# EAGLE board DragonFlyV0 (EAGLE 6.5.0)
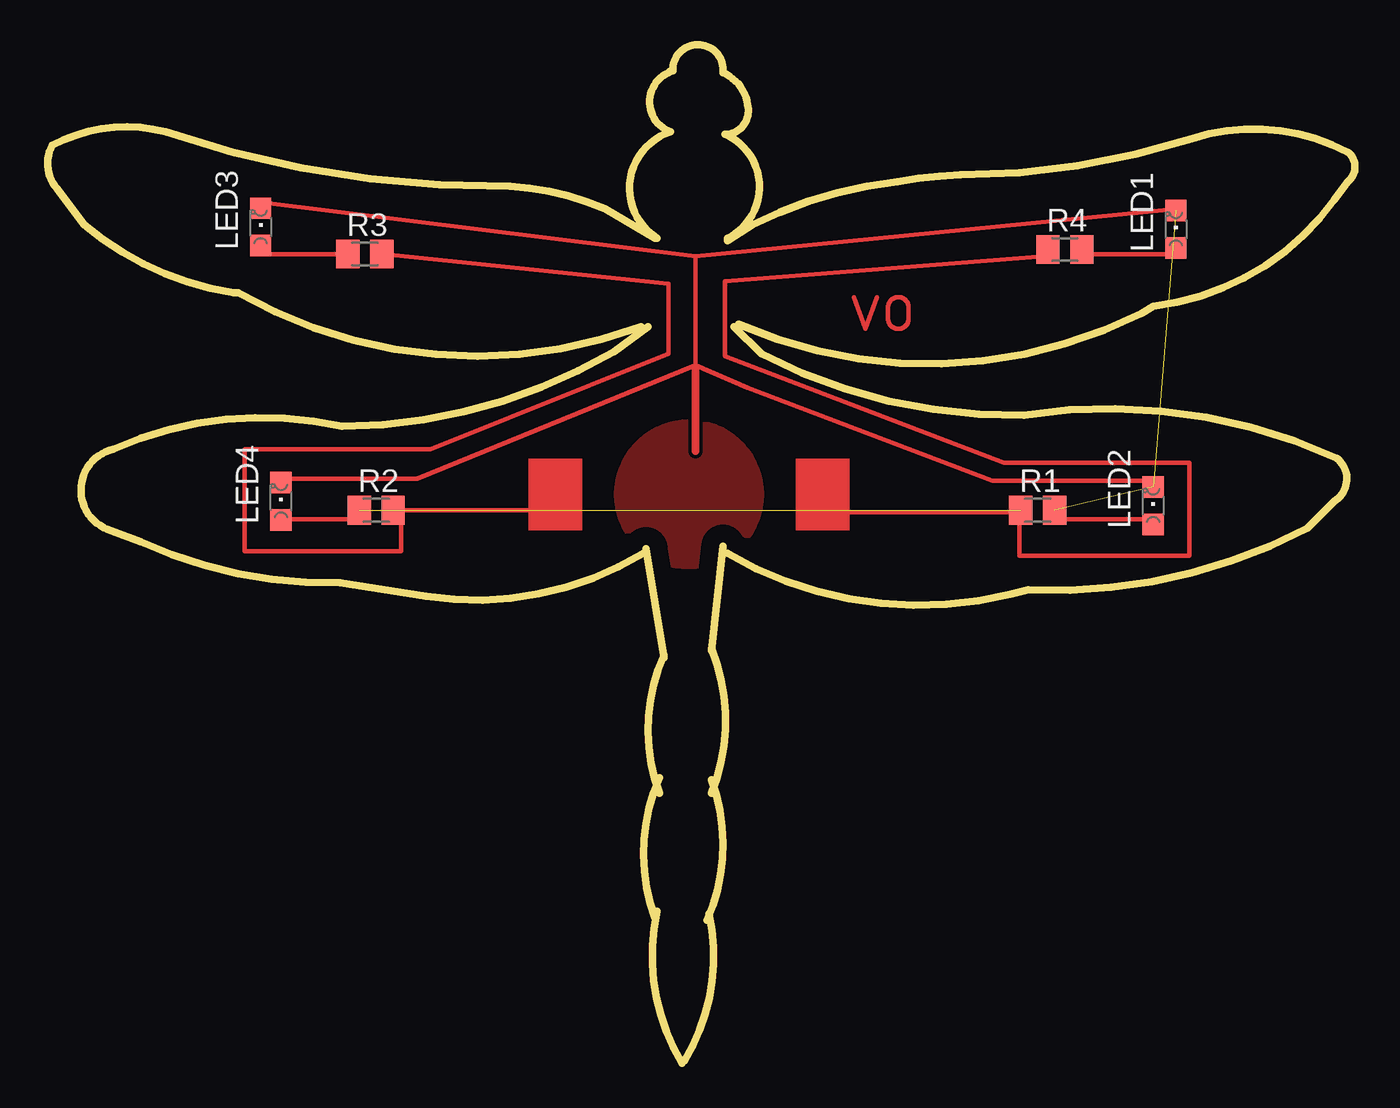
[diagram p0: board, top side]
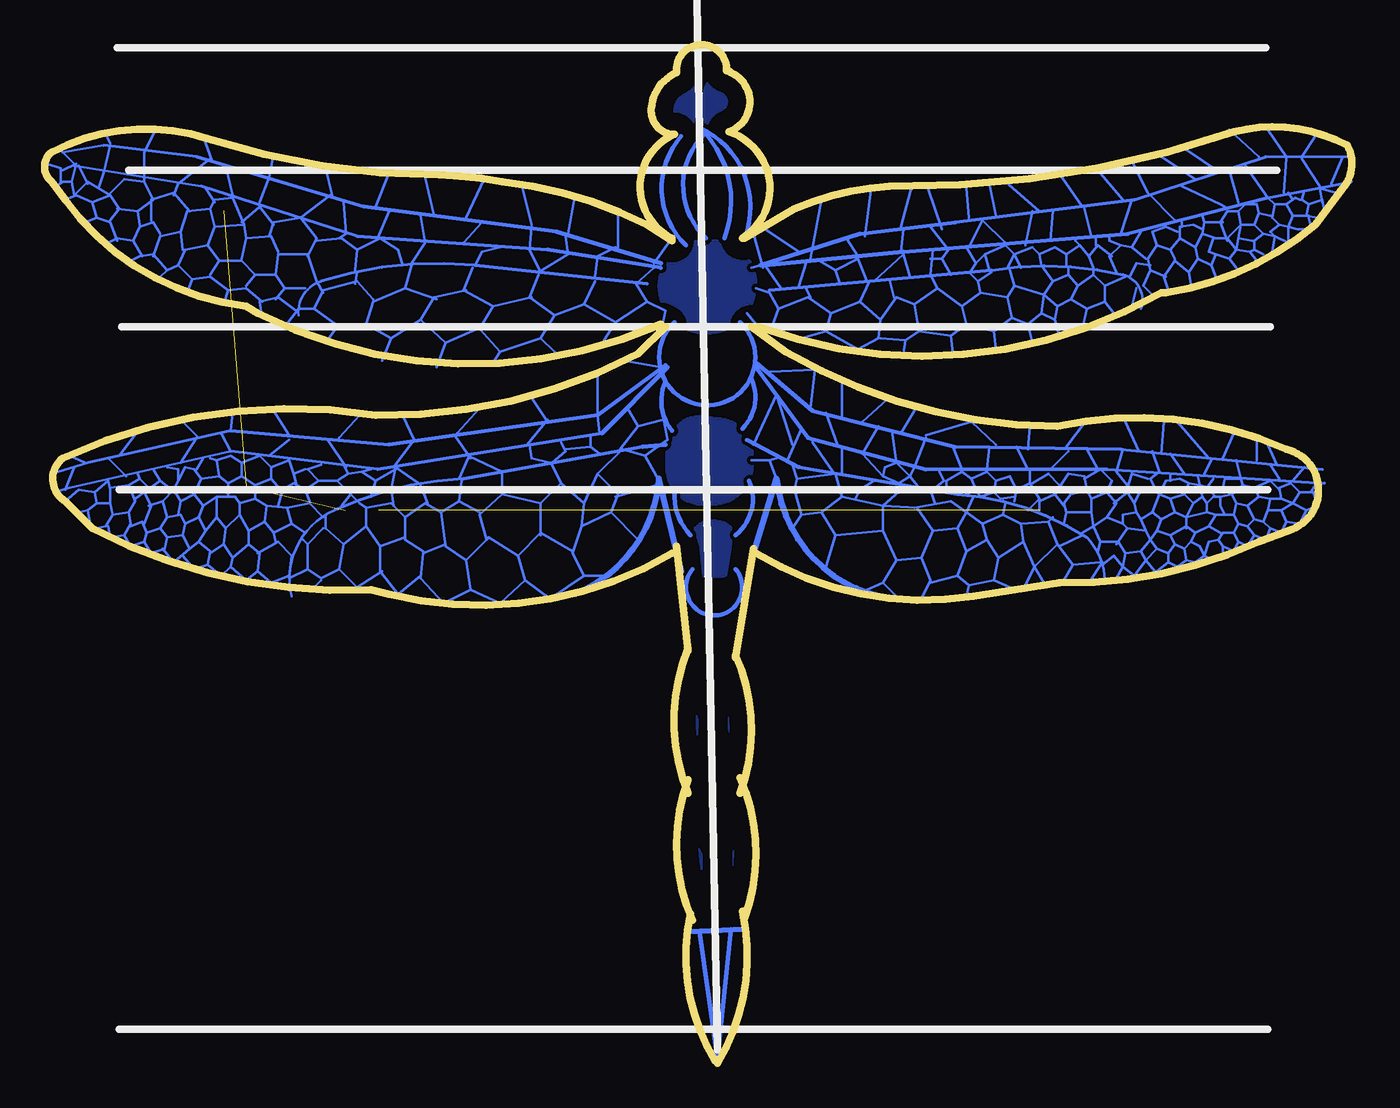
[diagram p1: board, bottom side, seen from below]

Size 73.29 x 57.08 mm. Coordinates in mm from the lower left corner, seen from the top.
Outline: 51 segments
Copper layers (1*16): Top 0.035mm / dielectric 1.5mm / Bottom 0.035mm
Design rules "default": minimum track width 10mil, minimum drill 24mil, track to track 8mil, track to pad 8mil, pad to pad 8mil, via to via 8mil, smd to smd 8mil, copper to edge 40mil, drill to drill 8mil, minimum pad ring 10mil, minimum via ring 8mil, stop-mask expansion 4mil, vias tented up to drill 0mil, thermal gap 10mil

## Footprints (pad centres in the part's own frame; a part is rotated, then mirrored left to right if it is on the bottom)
CHIPLED_0805 = smd 1.2 x 1.2: A 0,-1.05; C 0,1.05
M0805 = smd 1.3 x 1.6: 1 -0.95,0; 2 0.95,0

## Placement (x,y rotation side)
LED1  [CHIPLED_0805]  63.26,46.74 0 top
LED2  [CHIPLED_0805]  61.99,31.24 0 top
LED3  [CHIPLED_0805]  11.95,46.86 0 top
LED4  [CHIPLED_0805]  13.09,31.5 0 top
R1  [M0805]  55.51,30.99 0 top
R2  [M0805]  18.42,30.99 0 top
R3  [M0805]  17.79,45.34 0 top
R4  [M0805]  57.03,45.59 0 top

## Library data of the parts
LED1-LED4 = led
R1-R4 = resistor

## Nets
N$1: LED2.A
N$2: LED1.C LED2.C R1.2
N$6: R1.1 R2.1

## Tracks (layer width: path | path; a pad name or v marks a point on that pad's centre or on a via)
N$2  (2 unrouted)
N$3
  Bottom 0.127: 32.27,32.77 32.65,33.78 | 32.65,33.78 32.27,33.91 | 32.65,33.78 33.66,33.78
  Bottom 0.33: 33.66,28.19 32.27,32.77
N$4
  Bottom 0.33: 38.87,32.77 37.6,27.56
N$5
  Bottom 0.127: 66.05,48.64 65.8,49.28 64.02,50.67
N$6  (1 unrouted)
N$7
  Bottom 0.127: 42.43,44.07 42.3,45.21 41.28,45.72
N$8
  Bottom 0.127: 71.51,50.29 72.27,51.05 | 72.27,51.05 72.4,51.18 | 69.99,51.44 72.27,51.05
  Bottom 0.178: 64.78,50.8 69.99,51.44
  Bottom 0.203: 55.38,48.01 64.78,50.8
  Bottom 0.229: 44.59,46.61 55.38,48.01
  Bottom 0.254: 38.74,44.83 44.59,46.61
N$9
  Bottom 0.152: 64.53,49.15 71.64,50.29
  Bottom 0.178: 55.76,46.35 64.53,49.15
  Bottom 0.203: 45.09,45.59 55.76,46.35
  Bottom 0.229: 38.74,44.58 45.09,45.59
N$10
  Bottom 0.127: 49.16,44.7 48.78,45.47 47.76,45.72
  Bottom 0.152: 57.79,43.81 arc-77 59.06,41.91
  Bottom 0.178: 49.16,44.7 arc-24 57.79,43.81
  Bottom 0.203: 39.51,43.69 49.16,44.7
N$11
  Bottom 0.127: 41.16,45.72 41.16,47.75
N$12
  Bottom 0.127: 43.95,46.48 43.57,48.51
N$13
  Bottom 0.127: 45.98,46.99 46.49,49.02
N$14
  Bottom 0.127: 49.67,47.37 48.65,49.53
N$15
  Bottom 0.127: 51.44,47.5 51.95,49.66
N$16
  Bottom 0.127: 54.75,48.01 53.98,49.91
N$17
  Bottom 0.127: 57.16,48.64 57.54,50.16
N$18
  Bottom 0.127: 60.46,50.93 60.72,49.66 61.22,48.26
N$19
  Bottom 0.127: 63.89,50.55 64.4,51.94
N$20
  pour Bottom: 37.86,17.4 arc90 37.98,17.4 37.98,20.07 arc90 37.73,19.94 37.35,19.94 arc90 36.71,18.8 36.71,18.54 arc90
N$21
  Bottom 0.127: 69.61,51.56 69.86,52.07
N$22
  Bottom 0.127: 45.6,44.32 43.95,45.34 44.08,46.35
N$23
  Bottom 0.127: 45.98,42.93 48.14,42.42 | 48.14,42.42 48.9,41.15 47.76,39.88 | 39.51,42.67 40.14,43.69 39.13,44.58 | 39.51,42.67 41.28,41.53 | 41.28,41.53 43.06,42.55 | 43.06,42.55 42.43,43.81 | 43.06,42.55 44.71,41.91 | 44.71,41.91 46.11,42.93 45.6,44.2 | 41.28,41.53 41.92,40.51 | 44.71,41.91 45.48,40.64 | 45.48,40.64 44.71,39.88 | 47.76,39.88 45.48,40.64 | 48.14,42.42 49.79,43.31 49.29,44.58 | 47.76,39.88 48.14,39.24 | 39.51,42.67 38.49,42.16 38.62,41.53
N$24
  Bottom 0.127: 45.48,44.32 46.11,45.59 45.98,46.86
N$25
  Bottom 0.127: 51.32,42.8 53.1,43.43 | 53.1,43.43 52.71,44.7 | 53.1,43.43 54.87,42.67 55.25,41.4 53.86,40.64 | 49.67,43.31 51.44,42.93 52.21,41.66 | 52.21,41.66 50.81,40.39 | 50.81,40.39 49.03,41.15 | 53.86,40.64 52.21,41.66 | 50.81,40.39 51.32,38.99 51.32,39.12 | 53.86,40.64 54.37,39.37
N$26
  Bottom 0.127: 55.13,41.4 56.91,41.27 57.54,40.39
N$27
  Bottom 0.127: 56.78,41.27 58.18,42.29 | 58.18,42.29 59.06,42.29 59.83,41.27 | 58.18,42.29 57.67,43.31 55.76,43.81 54.87,42.8
N$28
  Bottom 0.127: 55.89,43.69 55.76,44.32
N$29
  Bottom 0.127: 58.56,45.21 58.05,46.23 58.94,47.37 | 58.94,47.37 60.46,47.12 60.72,46.35 | 58.94,47.37 57.29,48.64
N$30
  Bottom 0.127: 59.19,42.16 60.21,42.93 61.22,42.67 61.1,41.78
N$31
  Bottom 0.127: 60.46,46.99 61.22,48.01 62.24,47.12
N$32
  Bottom 0.127: 63.76,48.26 64.27,49.02
N$33
  Bottom 0.127: 69.22,46.1 69.61,47.12 70.37,47.37 | 70.37,47.37 71,47.12 | 70.37,47.37 70.62,48.26 | 70.62,48.26 71.51,48.64 72.15,48.39 | 70.62,48.26 69.61,48.64 | 69.61,48.64 69.1,47.88 69.61,47.24 | 69.61,48.64 70.88,49.4 71.64,48.64 71.76,49.4 | 72.27,50.04 71.51,50.42 71.76,49.4 | 71.76,49.4 72.27,49.4 72.65,49.15
N$34
  Bottom 0.127: 62.75,48.64 63.13,50.29
N$35
  Bottom 0.127: 72.4,49.4 72.4,50.16 73.16,50.42
N$36
  pour Bottom: 33.54,10.54 34.05,10.54 arc90 34.68,11.18 34.68,11.56 arc90 33.54,12.7
N$37
  Bottom 0.127: 56.78,46.23 56.4,46.48 56.52,48.26
N$38
  Bottom 0.127: 66.81,46.48 67.19,47.12 67.95,46.86 68.34,46.1 | 67.83,45.21 68.34,46.1 | 68.34,46.1 69.22,46.23 69.73,45.97
N$39
  Bottom 0.127: 53.22,44.7 53.48,45.59 54.49,46.23 55.76,45.59 | 55.89,44.45 55.76,45.59 | 55.76,45.59 56.65,46.23 58.05,46.1
N$40
  pour Bottom: 33.66,14.1 34.17,14.1 arc90 35.19,15.11 35.19,15.88 arc90 34.43,16.64 33.92,16.64 arc90 33.79,16.51 34.05,15.49
N$41
  Bottom 0.127: 67.95,46.99 68.08,47.75 | 68.08,47.75 69.22,47.88 | 68.08,47.75 67.19,48.39 67.7,49.4 | 67.7,49.4 68.84,49.53 69.73,48.64 | 67.07,52.32 67.7,51.05 67.7,49.4
N$42
  Bottom 0.127: 70.88,49.28 71.38,50.29
N$43
  Bottom 0.127: 60.21,45.47 60.59,46.35 61.99,46.23 | 61.99,46.23 62.24,45.09 | 61.99,46.23 62.11,46.99 | 62.11,46.99 63.76,46.86 | 57.67,43.18 58.05,43.81 58.56,45.34 60.21,45.34 60.33,44.2 | 58.68,43.43 59.83,43.43 | 59.83,43.43 60.33,42.8 | 59.83,43.43 60.33,44.2 | 60.33,44.2 61.48,44.2 | 61.48,44.2 61.99,43.56 | 61.48,44.2 62.24,44.96 63.51,44.96 | 63.51,44.96 64.02,44.2 | 63.51,44.96 64.14,45.85 | 64.14,45.85 65.41,45.59 65.8,44.7 | 61.1,42.67 61.99,43.43 63,43.31 | 63,43.31 63.26,42.55 | 63,43.31 64.02,44.07 65.03,43.94 | 65.03,43.94 65.29,43.18 | 65.03,43.94 65.8,44.7 | 65.8,44.7 66.43,44.45 | 66.43,44.45 66.81,44.07 | 66.43,44.45 67.19,45.34 67.95,45.21 68.46,44.96 | 63.76,46.86 64.14,45.85 | 63.76,46.86 64.02,47.88 | 64.02,47.88 65.29,47.75 65.67,46.61 | 67.19,45.21 66.81,46.35 65.67,46.61 | 65.67,46.61 65.54,45.59 | 62.11,46.99 62.75,48.51 63.76,48.39 64.02,47.88
N$44
  Bottom 0.127: 65.16,47.75 66.05,48.77 67.32,48.39 67.32,47.24
N$45
  Bottom 0.127: 70.24,49.15 69.99,49.91 69.61,51.44
N$46
  pour Bottom: 34.93,55.63 arc-90 36.33,54.1 36.33,53.21 arc-90 35.44,52.2 arc-167 35.06,55.63
N$47
  pour Bottom: 37.98,55.5 arc90 36.71,53.98 36.71,53.59 arc90 37.98,52.07 arc100 39.25,53.59 arc47
N$48
  pour Bottom: 33.79,20.32 33.92,20.32 arc-90 34.93,19.3 34.93,18.92 arc-90 33.79,17.78
N$49
  pour Bottom: 37.86,10.29 37.98,12.45 37.6,12.45 37.47,12.45 arc90 36.46,11.43 36.46,11.05 arc90 36.84,10.67
N$50
  pour Bottom: 37.98,13.21 37.47,15.75 arc90 36.46,14.73 36.46,14.48 arc90 37.73,13.21
N$51
  Bottom 0.127: 36.59,7.37 37.22,7.37
  Bottom 0.254: 34.81,7.49 35.57,0.25 36.59,7.37
  Bottom 0.305: 37.22,7.37 34.05,7.49
N$52
  Bottom 0.33: 38.87,32.64 arc63 43.57,26.29
N$53
  Bottom 0.33: 32.27,32.77 arc-71 26.43,26.16
N$54
  Bottom 0.127: 54.62,46.23 53.98,47.75
N$55
  Bottom 0.127: 52.71,44.83 51.95,45.97 52.21,47.5
N$56
  Bottom 0.127: 48.78,47.12 49.79,45.97
N$57
  Top 0.254: 44.71,30.86 54.37,30.86
N$58
  Top 0.254: 56.78,30.48 61.99,30.48
N$59
  Top 0.254: 54.49,30.73 54.49,28.45 64.02,28.45 64.02,33.66 53.6,33.66 37.98,39.62 37.98,43.81 55.89,45.21 55.64,45.21
N$60
  Top 0.254: 58.3,45.34 63.38,45.34
N$61
  Top 0.254: 63.38,47.88 36.33,45.21 36.33,38.99
  Top 0.406: 36.33,38.99 36.33,34.29
N$62
  Top 0.254: 62.11,32.64 52.97,32.64 39.25,37.85 36.33,39.12
N$63
  Top 0.254: 27.82,30.99 19.44,30.99
N$64
  Top 0.254: 17.41,30.48 13.22,30.48
N$65
  Top 0.254: 13.09,32.77 20.71,32.77 36.33,39.12
N$66
  Top 0.254: 19.82,30.86 19.82,28.7 11.06,28.7 11.06,34.42 21.47,34.42 34.81,39.75 34.81,43.69 18.93,45.34
N$67
  Top 0.254: 16.65,45.34 12.07,45.34
N$68
  Top 0.254: 11.95,48.26 36.33,45.21
N$69
  Bottom 0.127: 33.16,44.7 33.66,44.58 | 1.15,49.28 0.52,50.8 0.01,50.8 | 2.8,50.8 2.04,51.94 | 3.69,50.8 4.71,52.32
  Bottom 0.152: 4.84,50.8 3.69,50.8 2.8,50.8 0.52,50.8
  Bottom 0.178: 12.2,48.39 4.84,50.8
  Bottom 0.203: 22.23,47.12 12.2,48.39
  Bottom 0.229: 27.57,46.48 22.23,47.12
  Bottom 0.254: 33.16,44.7 27.57,46.48
N$70
  Bottom 0.127: 55,31.75 54.75,32.64 | 54.75,32.64 55.51,33.15 | 57.79,33.53 58.56,33.27 57.92,32.64 | 56.65,31.24 56.14,31.88 | 56.14,31.88 56.91,32.64 | 56.91,32.64 57.92,32.64 | 57.92,32.64 58.68,32.13 | 58.68,32.13 58.43,31.5 | 58.68,32.13 59.32,32.51 59.95,32.13 60.21,31.24 | 56.91,32.64 56.27,33.02 | 56.27,33.02 56.52,33.53 | 57.67,29.97 58.56,29.08 | 58.56,29.08 58.81,29.34 | 58.56,29.08 58.56,27.69 | 58.56,27.69 57.79,27.18 56.78,27.69 | 54.37,27.56 55.76,26.67 56.78,27.69 | 56.78,27.69 56.52,29.08 | 56.52,29.08 55.25,30.1 | 52.21,27.3 53.48,26.29 54.49,27.56 54.49,28.96 | 52.08,28.7 53.1,29.34 53.1,29.46 | 53.1,29.46 53.1,30.61 | 53.1,30.61 51.95,31.37 51.06,30.86 | 39,32.89 39.63,34.04 | 39.63,34.04 40.9,34.42 42.3,33.02 | 43.7,28.7 45.48,29.72 46.75,28.45 | 46.75,28.45 46.36,27.05 | 46.36,27.05 44.97,26.04 43.06,27.3 | 40.01,29.34 41.54,30.86 | 41.54,30.86 43.19,30.1 | 43.19,30.1 43.7,28.57 43.06,27.3 | 43.06,27.3 41.79,27.3 | 46.36,27.05 47.76,25.78 49.41,26.54 | 49.41,26.54 49.67,28.19 | 49.67,28.19 48.52,29.34 | 48.52,29.34 48.4,29.46 46.75,28.45 | 48.52,29.34 48.9,30.73 47.63,31.88 45.48,31.37 | 45.48,31.37 45.48,29.59 | 43.19,30.1 43.06,31.37 | 43.06,31.37 44.33,32.51 | 44.33,32.51 45.48,31.37 | 41.54,30.86 41.16,31.88 42.3,33.02 | 42.3,33.02 43.06,31.37 | 44.33,32.51 44.84,33.53 | 49.67,28.19 50.81,28.96 51.06,30.86 | 48.9,30.86 50.05,31.5 | 50.05,31.5 49.92,32.64 | 51.06,30.86 50.05,31.5 | 49.41,26.54 50.94,25.78 52.21,27.18 52.08,28.57 50.81,29.08 | 54.49,28.96 53.1,29.46 | 55.25,30.1 54.49,28.96 | 53.1,30.61 53.73,31.24 | 53.73,31.24 53.86,31.37 55.25,31.12 | 55.25,31.12 55.25,30.1 | 53.73,31.24 53.86,32.26 | 55.25,31.12 55.64,31.37 56.14,31.88
  Bottom 0.127: 56.52,29.08 57.54,29.97 57.54,30.73 | 58.56,27.69 59.57,27.18 | 55.51,33.15 56.27,33.02 | 55.51,33.15 55,33.27 | 54.75,32.64 53.6,33.27 | 39.63,34.04 38.36,34.92 38.74,36.83
  Bottom 0.152: 57.03,30.99 arc-80 59.45,26.16
  Bottom 0.178: 49.79,32.77 arc-21 57.03,30.99
  Bottom 0.203: 39.76,34.54 49.79,32.77
  Bottom 0.254: 39.76,34.54 38.49,34.67
N$71
  Bottom 0.152: 12.84,44.2 arc93 11.82,42.29
  Bottom 0.178: 20.2,44.45 arc22 12.84,44.2
  Bottom 0.203: 32.65,43.31 20.2,44.45
N$72
  Bottom 0.127: 42.3,38.61 42.3,36.32 42.17,35.31 | 62.87,35.43 62.75,36.45 | 69.73,33.91 68.72,32.89 | 70.88,33.66 72.91,33.02
  Bottom 0.178: 62.87,35.43 69.73,33.91 70.88,33.66
  Bottom 0.203: 53.98,34.67 62.87,35.43
  Bottom 0.229: 42.3,36.32 53.98,34.67
  Bottom 0.254: 38.49,39.12 42.3,36.32
N$73
  Bottom 0.127: 62.87,34.29 63.38,35.31 | 71.89,32.26 72.78,32
  Bottom 0.152: 62.87,34.29 71.89,32.26
  Bottom 0.178: 54.62,33.27 62.87,34.29
  Bottom 0.203: 42.05,35.31 54.62,33.27
  Bottom 0.254: 38.36,38.99 42.05,35.31
N$74
  Bottom 0.127: 41.03,34.42 40.01,35.69 | 40.01,35.69 40.52,36.58 | 40.01,35.69 38.62,36.07
N$75
  Bottom 0.127: 38.74,38.99 40.78,39.37
N$76
  Bottom 0.127: 46.11,37.46 45.09,35.94
N$77
  Bottom 0.127: 48.9,36.7 50.17,35.31
N$78
  Bottom 0.127: 53.22,36.32 52.59,34.92 53.73,33.4
N$79
  Bottom 0.127: 55.64,36.32 56.78,35.05
N$80
  Bottom 0.127: 59.57,35.18 60.46,36.58
N$81
  Bottom 0.127: 64.65,35.05 65.54,35.94
N$82
  Bottom 0.127: 67.95,35.56 69.1,34.04
N$83
  Bottom 0.127: 45.09,36.07 46.24,34.67
N$84
  Bottom 0.127: 49.41,33.91 50.3,35.18
N$85
  Bottom 0.127: 56.4,33.4 57.41,34.92
N$86
  Bottom 0.127: 59.57,34.92 60.72,34.04
N$87
  Bottom 0.127: 64.78,35.05 65.67,33.66
N$88
  Bottom 0.127: 42.17,34.16 42.68,34.54 | 42.68,34.54 42.68,35.18 | 42.68,34.54 44.08,34.42
N$89
  Bottom 0.127: 39.13,44.83 38.24,46.1
N$90
  Bottom 0.127: 59.19,32.51 59.32,33.02 | 59.32,33.02 58.68,33.27 | 59.32,33.02 59.57,33.78 60.59,33.4 | 59.95,32 60.59,32.77 | 60.59,32.77 61.48,32.38 | 67.45,32.26 67.95,32.77 | 57.67,30.61 58.43,31.37 59.7,31.12 | 58.68,29.72 59.45,30.23 | 59.45,30.23 60.46,29.72 | 60.46,29.72 60.33,29.21 | 60.46,29.72 60.97,30.35 | 60.97,30.35 61.86,29.84 | 64.02,28.57 63.26,29.08 | 63.26,29.08 62.75,28.32 | 62.75,28.32 62.87,27.81 | 62.87,27.81 63.38,27.3 64.14,27.94 | 68.46,30.1 67.83,30.35 67.57,29.72 | 67.57,29.72 67.7,29.21 | 67.7,29.21 68.46,28.96 68.84,29.59 | 72.15,31.5 71.38,32.13 70.49,32 | 70.49,32 70.37,31.37 | 70.37,31.37 70.88,30.99 | 70.88,30.99 71.38,30.86 | 70.75,30.23 70.88,30.99 | 70.37,31.37 69.61,31.37 | 69.61,31.37 69.48,30.73 | 69.48,30.73 69.86,30.1 70.37,29.97 | 69.48,30.73 68.59,30.86 | 68.59,30.86 68.46,30.23 68.84,29.59 | 68.84,29.59 69.61,29.46 69.73,30.1 | 67.57,29.72 66.81,29.97 | 66.81,29.97 66.43,29.46 | 66.43,29.46 66.56,28.83 67.32,28.57 67.7,29.21 | 66.43,29.46 65.54,29.59 | 65.54,29.59 65.16,28.83 | 65.16,28.83 66.05,28.07 66.68,28.83 | 65.16,28.83 64.65,29.21 | 64.65,29.21 64.02,28.7 64.14,27.94 | 64.14,27.94 64.91,27.69 65.54,28.45 | 68.59,30.86 68.21,31.5 68.59,32.38 | 68.59,32.38 69.61,32.26 69.61,32.13 | 69.61,32.13 69.61,31.37 | 69.61,32.13 69.73,32.64 70.49,32 | 66.81,29.97 66.43,30.61 | 66.43,30.61 66.68,31.5 | 66.68,31.5 67.45,31.24 | 65.54,29.59 65.41,30.23 | 65.41,30.23 65.67,30.73 66.43,30.61 | 64.65,29.21 64.27,29.84 | 64.27,29.84 64.65,30.61 | 64.65,30.61 65.41,30.23 | 62.87,27.81 61.99,27.05 61.35,27.56 | 61.35,27.56 61.22,28.57 61.86,29.08 | 61.86,29.08 62.75,28.32 | 61.35,27.56 60.59,26.92 59.57,27.3 59.45,28.45 60.21,29.21 61.35,28.57
  Bottom 0.127: 61.86,29.84 61.86,29.08 | 63.26,29.08 63.13,29.97 | 63.13,29.97 62.37,30.73 | 62.37,30.73 61.86,29.84 | 63.13,29.97 63.64,30.61 | 63.64,30.61 64.27,29.84 | 59.7,31.12 59.45,30.23 | 59.7,31.12 60.84,31.24 | 60.84,31.24 60.97,30.35 | 60.84,31.24 61.48,31.62 | 61.48,31.62 62.37,31.37 | 62.37,31.37 62.37,30.73 | 62.37,31.37 62.62,31.75 63,31.75 | 63,31.75 63.64,31.75 | 63.64,31.75 63.64,30.61 | 64.65,30.61 64.4,31.24 | 64.4,31.24 63.64,31.75 | 64.4,31.24 64.91,31.88 | 64.91,31.88 65.67,31.5 | 65.67,31.5 65.8,30.73 | 65.67,31.5 66.05,32.13 | 66.05,32.13 66.68,31.5 | 67.95,32.77 68.59,32.38 | 67.95,32.77 68.08,33.02 | 61.48,32.38 61.48,31.62 | 61.48,32.38 62.24,32.89 | 62.24,32.89 63,32.51 | 63,32.51 63,31.75 | 63,32.51 63.51,32.89 | 63.51,32.89 64.53,32.77 | 64.53,32.77 64.91,31.88 | 64.53,32.77 64.91,33.27 65.41,33.4 65.8,32.64 | 65.8,32.64 66.05,32.13 | 65.8,32.64 65.8,33.27 66.43,33.4 | 60.59,33.4 60.59,32.77 | 60.59,33.4 61.22,34.04 62.24,33.66 | 62.24,33.66 62.24,32.89 | 62.24,33.66 62.87,34.04 63.64,33.78 | 63.64,33.78 63.51,32.89 | 63.64,33.78 64.02,33.91
N$91
  Bottom 0.127: 67.7,30.23 67.32,31.24 67.7,32 | 67.7,32 68.21,31.62 | 67.7,32 66.81,32.64 | 66.81,32.64 66.18,32.13 | 66.81,32.64 67.19,33.27
N$92
  Bottom 0.127: 64.78,33.27 64.4,33.91
N$93
  Bottom 0.127: 44.84,33.66 44.08,34.29 44.33,34.8
N$94
  Bottom 0.127: 39,32.38 41.28,31.75
N$95
  Bottom 0.127: 44.97,33.66 45.98,33.91 46.11,34.67
N$96
  Bottom 0.127: 47.63,32 47.63,33.02
N$97
  Bottom 0.127: 47.63,33.15 49.54,34.04
N$98
  Bottom 0.127: 25.66,42.93 25.92,43.94
N$99
  Bottom 0.127: 51.83,31.37 52.21,32.38
N$100
  Bottom 0.127: 30.36,42.93 30.62,43.43
N$101
  Bottom 0.127: 50.05,32.77 49.54,33.91
N$102
  Bottom 0.127: 52.33,32.51 53.6,33.4 53.86,32.13
N$103
  Bottom 0.127: 57.79,27.05 58.18,26.67
N$104
  Bottom 0.127: 33.41,41.4 33.92,42.04
N$105
  Bottom 0.127: 31,43.56 30.62,44.83
N$106
  Bottom 0.127: 27.7,45.21 28.33,46.23
N$107
  Bottom 0.127: 72.15,32.13 71.64,33.4
N$108
  Bottom 0.127: 71,33.66 71.89,34.04
N$109
  Bottom 0.127: 25.28,45.47 25.16,46.74
N$110
  Bottom 0.127: 23.63,46.86 22.74,45.72
N$111
  Bottom 0.127: 12.33,42.42 12.07,43.43
N$112
  Bottom 0.127: 21.47,45.72 20.71,47.24 19.44,45.97
N$113
  Bottom 0.127: 18.3,45.85 17.92,47.75
N$114
  Bottom 0.127: 2.42,47.37 2.3,46.86
N$115
  Bottom 0.127: 16.77,47.75 16.9,46.1
N$116
  Bottom 0.127: 0.9,48.77 1.79,49.02 1.66,48.26
N$117
  Bottom 0.127: 14.61,46.35 15,47.88
N$118
  Bottom 0.127: 12.96,46.48 12.33,48.39
N$119
  Bottom 0.127: 9.92,47.24 11.44,48.77 12.33,50.55
N$120
  Bottom 0.127: 3.31,48.39 3.57,48.77
N$121
  Bottom 0.127: 9.53,49.15 7.38,48.13 7.12,48.01
N$122
  Bottom 0.127: 6.36,48.26 6.87,50.04
N$123
  Bottom 0.127: 3.82,48.77 3.69,50.67
N$124
  Bottom 0.127: 2.8,50.67 1.79,49.15
N$125
  Bottom 0.127: 9.79,46.61 10.42,46.86 11.19,46.61 10.93,45.85 | 8.39,46.74 8.9,46.99 9.66,46.86 9.66,46.23 | 11.19,43.05 11.69,43.56 11.31,44.45 | 11.31,44.45 10.42,44.07 | 11.31,44.45 11.44,45.09 10.93,45.85 | 10.93,45.85 10.17,45.59 | 10.17,45.59 9.92,45.09 9.92,44.96 | 10.3,43.31 10.55,44.07 9.92,44.96 | 9.03,43.69 9.15,44.32 | 9.15,44.32 8.65,45.09 | 7.25,47.12 8.26,47.12 | 8.26,47.12 8.39,46.48 | 7.63,44.07 7.88,44.7 | 7.88,44.7 7.63,45.34 | 5.34,44.96 5.72,45.47 | 5.72,45.47 6.49,45.59 | 6.49,45.59 6.87,45.09 | 6.87,45.09 6.49,44.58 | 5.6,46.1 6.36,46.23 | 6.36,46.23 6.23,46.99 | 2.42,47.5 3.31,47.5 | 3.31,47.5 3.57,46.86 | 3.57,46.86 3.06,46.74 2.68,46.74 | 3.57,46.86 3.57,45.97 4.33,46.35 | 3.57,46.86 4.07,46.99 | 4.07,46.99 4.58,46.61 4.33,46.35 | 4.45,45.47 4.33,46.35 | 4.33,46.35 4.96,46.48 | 4.96,46.48 5.47,46.1 5.47,45.59 | 5.47,45.59 4.96,45.34 | 3.31,47.5 3.69,48.13 | 3.69,48.13 3.18,48.51 2.93,48.39 2.8,48.39 | 1.53,47.62 1.66,48.39 2.42,48.13 | 2.42,48.13 2.55,47.5 1.91,47.37 | 2.42,48.13 2.8,48.39 | 2.8,48.39 2.68,48.89 | 4.07,46.99 4.45,47.37 4.33,48.13 | 4.33,48.13 3.69,48.13 | 4.96,46.48 5.47,46.99 | 5.47,46.99 5.22,47.62 | 5.22,47.62 4.58,47.5 | 6.23,46.99 5.47,46.99 | 6.49,45.59 6.36,46.23 | 7.63,45.34 6.87,45.09 | 6.49,45.59 6.99,46.23 | 6.99,46.23 7.63,46.23 | 7.63,46.23 7.76,46.23 8.01,45.47 7.63,45.34 | 6.23,46.99 6.99,46.23 | 6.23,46.99 6.36,47.75 | 6.36,47.75 6.99,47.75 7.38,47.12 6.99,46.1 | 8.39,46.48 7.63,46.23 | 5.22,47.62 5.34,48.13 5.98,48.13 6.36,47.75 | 4.33,48.13 4.71,48.51 5.98,50.29 | 8.65,45.09 7.88,44.7 | 5.47,45.59 5.72,45.47 | 9.92,44.96 9.15,44.32 | 8.65,45.09 8.77,45.72 | 8.77,45.72 8.39,46.48 | 10.17,45.59 9.66,46.23
  Bottom 0.127: 9.66,46.23 8.77,45.72 | 8.26,47.12 8.39,47.5 | 32.01,43.43 32.9,44.7
  Bottom 0.178: 4.71,48.51 0.01,49.4
  Bottom 0.203: 12.58,46.48 4.71,48.51
  Bottom 0.229: 25.16,45.47 12.58,46.48
  Bottom 0.254: 32.9,44.7 25.16,45.47
N$126
  Bottom 0.127: 9.53,46.86 9.53,47.12
N$127
  Bottom 0.127: 12.46,44.07 12.07,44.83 11.31,44.7
N$128
  Bottom 0.254: 34.05,46.23 arc-86 36.59,52.45 arc68 35.19,46.23
N$129
  Bottom 0.127: 13.22,44.32 13.6,45.21 12.96,45.85 | 11.57,45.09 12.33,45.72 | 12.33,45.72 11.82,46.61 | 12.96,45.85 12.33,45.72 | 12.96,45.85 13.6,46.1 13.6,46.35
N$130
  Bottom 0.254: 37.6,51.94 arc-87 37.35,45.85
N$131
  Bottom 0.127: 14.36,45.85 14.36,46.35
N$132
  Bottom 0.127: 21.35,44.45 21.09,44.83 | 21.09,44.83 21.6,45.72 | 14.49,44.58 14.74,45.21 | 14.74,45.21 14.23,45.85 13.47,45.21 | 14.74,45.21 15.25,45.85 | 15.25,45.85 16.01,45.34 | 16.01,45.34 16.01,44.7 | 15.25,45.85 15.5,46.1 | 16.01,45.34 16.65,45.72 17.54,45.34 | 13.34,42.04 13.85,42.67 | 16.39,40.77 16.65,41.66 | 16.65,41.66 17.41,42.04 | 17.92,40.39 18.17,41.4 | 19.95,40.01 20.08,41.02 | 22.36,39.75 22.49,40.77 | 25.16,39.75 25.03,40.51 | 25.03,40.51 26.43,40.64 | 25.03,40.51 24.27,41.02 | 24.27,41.02 24.52,42.55 | 24.52,42.55 25.54,42.93 26.43,41.66 | 32.52,41.27 32.14,42.29 | 32.14,42.29 30.49,42.93 29.22,42.04 | 29.22,42.04 29.47,41.02 | 29.47,41.02 30.87,40.64 | 29.22,42.04 27.57,42.67 | 27.57,42.67 26.43,41.66 | 26.43,41.66 26.55,40.64 27.7,40.01 29.47,41.02 | 22.49,40.77 24.27,41.02 | 22.49,40.77 21.6,41.4 | 21.6,41.4 21.85,42.42 | 21.85,42.42 23.25,43.43 | 23.25,43.43 24.52,42.55 | 27.57,42.67 27.06,43.81 | 23.25,43.43 23.63,44.2 23.5,45.59 | 20.08,41.02 21.6,41.4 | 20.08,41.02 19.06,41.78 | 19.06,41.78 19.31,42.93 | 19.31,42.93 20.84,43.18 | 20.84,43.18 21.85,42.42 | 20.84,43.18 20.96,43.81 | 20.96,43.81 21.47,44.32 | 20.96,43.81 20.2,44.32 | 19.31,42.93 18.93,43.56 | 18.93,43.56 19.19,44.45 | 18.17,41.4 19.06,41.78 | 17.41,42.04 18.17,41.4 | 17.41,42.04 17.28,43.05 | 17.28,43.05 18.93,43.56 | 17.28,43.05 16.77,43.81 | 16.77,43.81 17.41,44.7 17.54,45.34 | 15.12,41.15 14.87,42.29 | 14.87,42.29 15.76,42.8 | 15.76,42.8 16.52,42.42 | 16.65,41.66 16.52,42.42 | 16.52,42.42 17.28,43.05 | 15.76,42.8 15.38,43.56 | 15.38,43.56 15.88,44.2 | 15.88,44.2 16.77,43.81 | 13.85,42.67 14.87,42.29 | 13.85,42.67 13.85,43.56 | 13.85,43.56 12.71,44.07 | 13.85,43.56 14.49,44.2 | 14.49,44.2 15.38,43.56
  Bottom 0.127: 14.49,44.2 14.49,44.45 | 15.88,44.2 15.88,44.58 | 17.54,45.34 17.92,45.72 18.93,45.34 | 18.93,45.34 18.55,44.58 | 19.31,44.58 18.93,45.34 | 18.93,45.34 19.44,45.85 20.58,45.34 | 20.58,45.34 20.33,44.45 | 21.09,44.83 20.58,45.34 | 32.14,42.29 32.65,43.18 33.41,43.43
N$133
  Bottom 0.127: 22.62,45.59 23,45.09 | 23,45.09 22.49,44.2 | 23,45.09 23.63,45.09
N$134
  Bottom 0.127: 24.77,44.07 25.16,45.34 26.81,43.81
N$135
  Bottom 0.127: 27.19,43.81 27.7,45.09 28.97,44.45 | 28.97,44.45 28.71,43.69 | 28.97,44.45 29.85,44.96
N$136
  pour Bottom: 33.41,43.69 arc-90 35.82,46.1 36.33,46.1 arc-90 38.87,43.56 arc-90 36.2,40.89 arc-90
N$137
  Bottom 0.254: 34.3,41.53 arc274 37.98,41.53
N$138
  pour Bottom: 35.57,36.07 arc90 33.66,34.04 33.66,33.53 arc90 35.82,31.37 36.33,31.37 arc90 38.36,33.27 38.36,34.54 arc90 36.33,36.2
N$139
  pour Bottom: 35.82,30.35 arc90 34.3,28.83 34.3,28.57 arc90 35.57,27.3 35.95,27.3 arc90 37.22,28.57 37.22,28.7 37.22,28.96 arc90
N$140
  Bottom 0.254: 34.55,27.69 arc260 36.97,27.69
N$141
  Bottom 0.254: 37.09,29.59 arc46 37.98,32
N$142
  Bottom 0.254: 38.11,35.43 arc63 38.49,38.23
N$143
  Bottom 0.254: 34.17,35.56 arc-69 33.66,38.35
N$144
  Bottom 0.254: 34.55,29.59 arc-74 33.79,32.64
N$145
  Bottom 0.254: 36.33,52.07 arc-91 36.2,46.23
N$146
  Bottom 0.127: 30.36,45.09 29.73,48.39
N$147
  Bottom 0.127: 33.03,44.58 33.54,46.48
N$148
  Bottom 0.127: 32.9,46.74 31,45.47
N$149
  Bottom 0.127: 27.31,46.35 26.93,49.15
N$150
  Bottom 0.127: 5.22,50.8 6.87,52.32
N$151
  Bottom 0.127: 7.38,49.91 9.28,51.18
N$152
  Bottom 0.127: 8.77,49.53 10.68,50.8
N$153
  Bottom 0.178: 12.96,34.42 1.66,33.27
  Bottom 0.203: 22.23,34.54 12.96,34.42
  Bottom 0.229: 30.24,36.58 22.23,34.54
  Bottom 0.254: 33.41,39.24 30.24,36.58
N$154
  Bottom 0.127: 12.84,48.39 14.23,50.04
N$155
  Bottom 0.127: 15.12,48.01 16.27,49.66
N$156
  Bottom 0.127: 19.95,47.5 20.33,49.28
N$157
  Bottom 0.127: 17.54,47.75 19.44,49.4
N$158
  Bottom 0.127: 21.47,47.37 21.6,49.02
N$159
  Bottom 0.127: 23,46.74 23.76,49.02
N$160
  Bottom 0.127: 31.38,34.67 32.27,37.46 33.54,34.67
N$161
  Bottom 0.127: 25.28,46.86 24.65,49.28
N$162
  Bottom 0.152: 14.87,29.46 arc43 13.85,27.05
  Bottom 0.178: 22.11,31.88 arc30 14.87,29.46
  Bottom 0.203: 31,33.4 22.11,31.88
  Bottom 0.229: 33.92,34.92 31,33.4
N$163
  Bottom 0.127: 30.87,30.73 31.25,32.13 32.14,32.26
N$164
  Bottom 0.127: 29.47,36.45 28.84,34.67
N$165
  Bottom 0.127: 28.97,29.59 29.73,30.86 30.87,30.73 31.38,29.97
N$166
  Bottom 0.127: 29.73,30.86 28.58,31.75 28.97,33.02 31.12,32.77 | 31.12,32.77 31.25,32.13 | 31.12,32.77 31.38,33.53
N$167
  Bottom 0.127: 7.38,29.72 8.01,30.1 | 4.07,32.13 4.58,32.64 5.47,32.26 | 13.22,27.18 12.84,27.81 | 12.84,27.81 13.34,28.45 13.98,27.94 | 12.84,27.81 12.2,27.3 11.57,28.19 | 12.84,27.81 12.71,28.57 | 12.71,28.57 11.82,28.7 | 11.82,28.7 11.57,28.19 | 11.06,27.56 11.57,28.19 | 11.57,28.19 10.93,28.83 | 10.93,28.83 10.3,28.57 | 10.3,28.57 10.3,28.07 | 10.3,28.07 10.93,27.56 | 10.3,28.07 9.79,27.81 9.28,28.19 | 9.28,28.19 9.41,28.83 | 9.41,28.83 9.92,29.08 | 9.92,29.08 10.3,28.57 | 9.28,28.19 8.77,28.07 8.26,28.45 | 8.26,28.45 8.52,28.96 9.03,29.21 | 9.03,29.21 9.41,28.83 | 8.26,28.45 7.76,28.19 7.25,28.45 7.25,28.96 | 8.26,28.45 8.01,29.21 7.5,29.34 | 7.5,29.34 7.25,28.96 | 7.25,28.96 6.61,28.7 6.36,29.21 | 7.5,29.34 7.25,29.72 6.61,29.72 | 6.61,29.72 6.36,29.21 | 6.36,29.21 5.85,28.96 5.47,29.59 | 5.47,29.59 5.85,30.1 | 5.85,30.1 6.36,30.23 | 6.36,30.23 6.61,29.72 | 5.47,29.59 4.84,29.34 4.58,29.97 | 4.58,29.97 4.96,30.35 | 4.96,30.35 5.47,30.48 | 5.47,30.48 5.85,30.1 | 4.58,29.97 3.95,29.72 3.69,30.35 | 3.69,30.35 3.95,30.99 | 3.95,30.99 4.71,30.99 | 4.71,30.99 4.96,30.35 | 3.69,30.35 2.93,30.23 2.55,30.99 | 3.95,30.99 3.31,31.37 | 3.31,31.37 2.55,30.99 | 2.55,30.99 1.91,31.24 2.17,32 2.3,32 | 2.3,32 2.93,32 | 2.93,32 3.31,31.37 | 2.93,32 3.44,32.51 4.07,32.26 3.95,31.62 | 2.3,32 2.04,32.38 | 3.31,31.37 3.95,31.62 | 3.95,31.62 4.58,31.62 | 4.58,31.62 4.71,30.99 | 4.58,31.62 5.22,31.75 | 5.22,31.75 5.85,31.24 | 5.85,31.24 5.47,30.48 | 5.47,32.26 5.22,31.75 | 12.71,28.57 13.09,29.21 14.11,29.21 | 14.11,29.21 14.23,28.7 | 10.93,28.83 11.31,29.34 | 11.31,29.34 11.82,28.7 | 9.92,29.08 10.17,29.59 | 10.17,29.59 10.93,29.84 | 10.93,29.84 11.31,29.34 | 11.31,29.34 11.57,29.84 | 11.57,29.84 12.58,29.97
  Bottom 0.127: 12.58,29.97 13.22,29.08 | 9.03,29.21 8.77,29.72 | 8.77,29.72 9.28,30.1 10.17,29.59 | 8.01,30.1 8.77,29.72 | 6.36,30.23 6.61,30.73 | 6.61,30.73 6.49,31.37 | 6.49,31.37 5.85,31.24 | 6.49,31.37 6.74,31.88 | 6.74,31.88 6.11,32.38 | 6.11,32.38 5.47,32.26 | 6.74,31.88 7.25,32.26 7.12,32.77 6.23,32.77 | 6.23,32.77 6.11,32.38 | 8.01,30.1 7.63,30.73 | 7.63,30.73 7.12,30.73 | 7.12,30.73 6.61,30.73 | 7.12,30.73 7.38,31.24 7.38,31.75 | 7.38,31.75 6.74,31.88 | 7.63,30.73 8.14,30.86 | 8.14,30.86 8.14,31.37 | 8.14,31.37 7.76,31.75 7.63,31.75 | 7.63,31.75 7.38,31.75 | 7.63,31.75 8.14,32.26 7.76,32.77 | 8.14,30.86 9.28,30.61 | 9.28,30.61 9.28,29.97 | 9.28,30.61 9.92,30.86 | 9.92,30.86 10.68,30.48 | 10.68,30.48 10.93,29.84 | 10.68,30.48 11.19,30.86 | 11.19,30.86 11.82,30.48 | 11.82,30.48 11.57,29.84 | 11.82,30.48 12.07,30.86 | 12.07,30.86 12.84,30.73 12.84,30.23 | 12.84,30.23 12.58,29.97 | 9.28,30.61 8.9,31.37 | 8.9,31.37 9.41,31.88 | 9.41,31.88 10.17,31.62 | 10.17,31.62 9.92,30.86 | 10.17,31.62 10.8,31.88 | 10.8,31.88 11.19,30.86 | 10.8,31.88 11.06,32.26 | 11.06,32.26 11.82,32.13 12.2,31.37 | 12.2,31.37 12.07,30.86 | 8.14,31.37 8.39,31.75 | 8.39,31.75 8.9,31.37 | 8.39,31.75 8.52,32.38 | 8.52,32.38 8.01,32.26 | 8.52,32.38 8.65,32.89 | 8.52,32.38 9.15,32.51 | 9.15,32.51 9.41,31.88 | 9.15,32.51 9.66,32.77 10.42,32.64 10.8,31.88 | 11.06,32.26 11.31,32.77 10.8,33.15 11.19,34.29 | 14.11,29.21 14.49,30.1 | 14.49,30.1 13.73,30.61 | 13.73,30.61 12.84,30.23 | 14.49,30.1 14.61,30.86 | 14.61,30.86 16.01,30.86 | 16.01,30.86 16.14,30.23 | 14.49,30.1 15.12,29.72 | 13.73,30.61 13.22,31.37 13.73,32 | 13.73,32 14.61,31.62 | 14.61,31.62 14.61,30.86 | 14.61,31.62 14.87,32.13 | 14.87,32.13 15.76,31.88 16.14,31.37 16.01,30.86
  Bottom 0.127: 14.87,32.13 15,32.89 15.88,33.02 16.65,31.88 | 16.14,31.24 16.65,31.88 | 16.65,31.88 17.54,31.5 17.54,30.99 | 13.73,32 13.47,32.64 14.11,33.27 15,32.77 | 12.2,31.37 12.58,32 13.34,31.37 | 22.36,34.54 21.85,33.27 | 20.46,33.27 20.33,34.54 | 18.17,33.27 18.81,34.54 | 16.9,33.27 15.88,34.29 | 14.23,33.27 14.87,34.42 | 6.49,33.78 6.23,32.77
  Bottom 0.178: 13.73,33.27 1.53,32.51
  Bottom 0.203: 23.89,33.27 21.85,33.27 20.46,33.27 18.17,33.27 16.9,33.27 14.23,33.27 14.11,33.27 13.73,33.27
  Bottom 0.229: 30.49,35.05 23.89,33.27
  Bottom 0.254: 33.41,38.99 30.49,35.05
N$168
  Bottom 0.127: 10.17,32.64 10.17,33.02
N$169
  Bottom 0.127: 23.38,31.37 23.63,32.13
N$170
  Bottom 0.127: 27.82,31.62 27.57,32.13 26.81,32.64
N$171
  Bottom 0.127: 16.14,27.05 15.63,27.94 | 15.63,27.94 16.52,29.08 | 18.3,26.8 17.79,27.81 | 17.79,27.81 18.42,29.21 | 23.63,26.92 22.11,27.3 | 22.11,27.3 21.6,28.7 | 21.6,28.7 22.11,29.97 | 24.14,26.04 23.63,27.05 24.14,28.32 | 29.47,27.81 28.97,29.59 26.3,29.84 | 26.3,29.84 25.54,28.19 | 25.54,28.19 26.3,26.92 | 26.3,26.92 27.44,26.42 | 26.3,26.92 25.54,26.16 | 24.14,28.32 25.54,28.19 | 24.14,28.32 23.5,29.84 | 23.5,29.84 24.39,31.12 26.3,31.24 | 26.3,29.84 26.3,31.24 | 26.3,31.24 28.58,31.75 | 26.3,31.24 25.16,32.26 | 22.11,29.97 23.5,29.84 | 22.11,27.3 21.47,26.8 | 21.47,26.8 21.6,26.16 | 21.47,26.8 20.08,27.05 | 20.08,27.05 19.82,28.32 | 19.82,28.32 20.46,29.34 | 20.46,29.34 21.6,28.7 | 20.08,27.05 19.19,26.67 | 18.42,29.21 19.82,28.32 | 18.42,29.21 18.55,30.23 | 18.55,30.23 19.57,30.73 | 19.57,30.73 20.71,30.23 | 20.71,30.23 20.46,29.34 | 20.71,30.23 21.6,30.86 | 21.6,30.86 22.11,29.97 | 21.6,30.86 22.49,31.5 24.52,31.12 | 21.6,30.86 21.22,31.75 | 16.52,29.08 17.79,27.81 | 17.79,27.81 17.28,26.92 | 16.52,29.08 17.03,30.35 | 17.03,30.35 18.55,30.23 | 19.57,30.73 19.44,31.37 | 17.03,30.35 16.77,30.61 | 15.63,27.94 14.11,28.07
N$172
  Bottom 0.127: 16.39,28.96 15.12,29.59
N$173
  Bottom 0.127: 13.98,28.07 14.74,26.92
N$174
  Bottom 0.127: 10.17,34.16 9.41,33.02
N$175
  Bottom 0.127: 8.26,33.02 7.88,33.78
N$176
  Bottom 0.127: 18.17,30.99 17.54,31.62 18.04,32.51 | 18.04,32.51 18.81,32.13 | 18.81,32.13 18.93,31.5 | 18.81,32.13 19.19,32.89 19.95,32.64 | 19.95,32.64 20.08,32 | 20.08,32 19.69,31.62 18.93,31.75 | 19.95,32.64 20.46,33.15 21.35,32.77 | 21.35,32.77 21.09,32.13 | 21.09,32.13 20.84,31.75 20.08,32 | 21.35,32.77 21.85,33.15 22.74,32.64 22.74,32 | 21.09,32.13 21.6,31.88 | 18.04,32.51 18.04,33.15
N$177
  Bottom 0.127: 23.5,32.13 22.87,32.64 23.12,33.15
N$178
  Bottom 0.127: 24.27,32.26 24.77,32.89 | 24.77,32.89 24.52,33.4 23.89,35.05 | 24.77,32.89 25.54,33.66 | 25.54,33.66 26.17,33.4 26.3,32.89 | 26.3,32.89 25.41,32.51 24.77,32.89 | 26.3,32.89 27.44,34.16 26.55,35.69 | 25.79,35.43 25.54,33.66
N$179
  Bottom 0.127: 16.39,32.38 17.03,33.02 17.92,32.51
N$180
  Bottom 0.127: 11.44,32.77 12.33,33.02 12.71,31.88
N$181
  Bottom 0.127: 12.58,32.38 13.22,33.15 12.84,34.42
N$182
  Bottom 0.127: 28.58,33.02 28.58,34.54
N$183
  Bottom 0.127: 30.24,34.8 29.09,33.15
N$184
  Bottom 0.127: 31.63,33.78 30.87,35.56
N$185
  Bottom 0.127: 4.07,32.77 4.58,33.53
N$186
  Bottom 0.127: 2.68,33.4 3.31,32.64
N$187
  Bottom 0.127: 30.36,36.7 30.11,38.86 32.65,38.73
N$188
  Bottom 0.127: 28.58,36.2 28.58,38.23
N$189
  Bottom 0.127: 27.44,35.94 26.04,37.21
N$190
  Bottom 0.127: 25.28,35.31 24.52,36.58
N$191
  Bottom 0.127: 4.2,33.53 4.71,34.67
N$192
  Bottom 0.127: 5.34,33.78 5.34,35.18
N$193
  Bottom 0.127: 7.25,33.91 6.61,35.31
N$194
  Bottom 0.127: 8.01,33.91 9.79,35.94
N$195
  Bottom 0.127: 10.68,34.16 10.55,35.94
N$196
  Bottom 0.127: 12.71,35.94 11.95,34.29
N$197
  Bottom 0.127: 16.01,34.54 14.87,36.07
N$198
  Bottom 0.127: 18.04,35.69 18.17,34.42
N$199
  Bottom 0.127: 19.95,34.67 21.35,35.94 23.89,35.18
N$200
  Top 0.254: 45.22,42.93 45.86,41.15 46.49,42.93
N$201
  Top 0.254: 47.13,42.42 arc-167 48.27,42.42 48.27,41.66 arc-167 47.13,41.66 47.13,42.42
S$1
  pour Top: 31.97,31.88 arc90 35.97,27.88 arc90 39.97,31.88 arc90 35.97,35.88 arc90
(copper drawn outside any net)
  shapes: Top area x2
